PROGRAM MAIN
VAR
	iCounter AT %Q* 		: UDINT;			// link to a digital/analogue output terminal
	iTest AT %I*	 		: UDINT;			// link to a digital/analogue input terminal

	(* ******************* EtherCAT Frame ***************************** *)
	fbEtherCATFrameDiag		: FB_EtherCATFrameDiag; // frame diagnostic 
	wFrmXWcState AT %I*		: WORD; 			// link to task related ethercat frame state (Frm1WcState)
	wReqZeroMask			: WORD := 16#FFFF; 	// clear bit to ignore datagram error of Frm1WcState
	bFrameWcStateOK			: BOOL;				// this frame is OK 
	bAllFrameWcStatesOK		: BOOL;				// all frames are OK

	(* ******************* EtherCAT Diag ***************************** *)
	fbEtherCATDiag			: FB_EtherCATDiag;	// deep EtherCAT diagnostic  
	bEtherCATOK				: BOOL;				// no problem on EtherCAT
	bFrameWcStateError		: BOOL;				// at least one fram with error
	bSlaveCountError		: BOOL;				// EtherCAT slave count mismatch (# of cfg slaves <> # of found slaves)
	bMasterDevStateError	: BOOL;				// EtherCAT master device state signals error
	stMasterDevState		: ST_EcMasterDevState; // device state split to a structure
	bBusy					: BOOL;				// diagnostic FB is busy
	bError					: BOOL;				// diagnostic FB has an error
	iErrorID				: UDINT;			// error ID of diagnostic FB

	(* cyclic variables from EtherCAT Master *)
	nEcMasterSlaveCount AT %I* 	: UINT;			// link to SlaveCount of EtherCAT Master (Inputs)
	nEcMasterDevState AT %I* 	: UINT;			// link to DevState of EtherCAT Master (Inputs)
	nEcMasterDeviceId AT %I*	: UINT;			// link to DevID of EtherCAT Master (InfoData)
	arrEcMasterNetId AT %I* 	: T_AmsNetIdArr;// link to NetID of EtherCAT Master (InfoData)
	sEcMasterNetId  			: T_AmsNetId := '';
	nEcMasterSlaveCountCfg AT %I* 	: UINT;		// link to CfgSlaveCount of EtherCAT Master (InfoData)

	(* general variables *)
	arrDiagSlaveInfo 			: ARRAY [0..3] OF ST_SlaveStateInfo;		// read in info of configured EtherCAT slaves 
	arrDiagSlaveInfoScanned		: ARRAY [0..3] OF ST_SlaveStateInfoScanned; // read in info of scanned EtherCAT slaves
END_VAR

iCounter := iCounter + 1;

(*************************************** Frame Diag *********************************************)
fbEtherCATFrameDiag(
	wFrmXWcState 	:= wFrmXWcState,
	wReqZeroMask 	:= wReqZeroMask,
	bFrameWcStateOK	=> bFrameWcStateOK
);
bAllFrameWcStatesOK := bFrameWcStateOK AND FAST.bFrameWcStateOK;

(*************************************** EtherCAT Diag *********************************************)
(* generate Net Id *)
sEcMasterNetId := F_CreateAmsNetId(nIds := arrEcMasterNetId);
fbEtherCATDiag(
	sIPCNetID			:= '',
	sMasterNetID		:= sEcMasterNetId,
	nMasterDevID		:= nEcMasterDeviceId,
	nSlaveCount			:= nEcMasterSlaveCount,
	nSlaveCountCfg		:= nEcMasterSlaveCountCfg,
	nMasterDevState		:= nEcMasterDevState,
	bAllFrameWcStatesOK	:= bAllFrameWcStatesOK,
	tTimeout			:= T#5s,
	arrDiagSlaveInfo	:= arrDiagSlaveInfo,
	arrDiagSlaveInfoScanned	:= arrDiagSlaveInfoScanned,
	bEtherCATOK			=> bEtherCATOK,
	bFrameWcStateError	=> bFrameWcStateError,
	bSlaveCountError	=> bSlaveCountError,
	bMasterDevStateError=> bMasterDevStateError,
	stMasterDevState	=> stMasterDevState,
	bBusy				=> bBusy,
	bError				=> bError,
	iErrorID			=> iErrorID
);

END_PROGRAM
